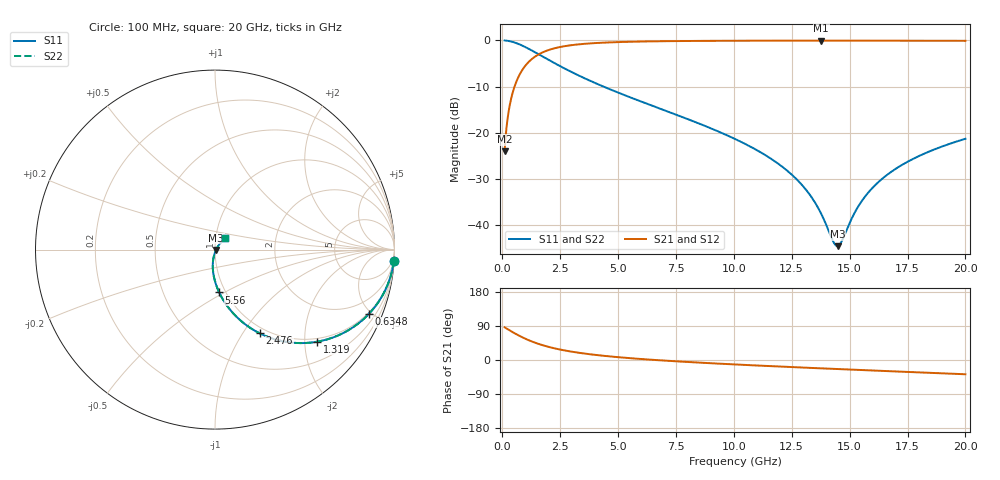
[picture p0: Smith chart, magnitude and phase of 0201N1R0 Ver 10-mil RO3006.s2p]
# GHz S MA R 50
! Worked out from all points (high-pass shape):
!   1601 points, 100 MHz to 20 GHz, reference 50 ohm
!   highest |S21| = -0.05 dB at 13.77 GHz (marker M1); lowest = -24.0 dB at 100 MHz (marker M2)
!   |S21| within 3 dB of the highest: 1.563 GHz to end of sweep
!   lowest |S11| = -44.6 dB at 14.48 GHz (marker M3), VSWR 1.01, Z = 50.5 - j0.238 ohm
!   |S11| at or under -10 dB: 4.364 GHz to end of sweep
!   |S22| runs from -44.6 to 0.0 dB; largest |S21 - S12| = 0
!   S11 on the Smith chart (normalised r, x): 100 MHz: 1, -30; 634.8 MHz: 0.92, -4.78; 1.319 GHz: 0.92, -2.29; 2.476 GHz: 0.92, -1.19; 5.56 GHz: 0.93, -0.47; 20 GHz: 1.11, +0.14
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0.1  0.998 -3.8  0.06274 86.2  0.06274 86.2  0.998 -3.8
0.3363125  0.9782 -12.5  0.2069 77.5  0.2069 77.5  0.9782 -12.5
0.6348125  0.9282 -22.8  0.3711 67.1  0.3711 67.1  0.9282 -22.8
0.9333125  0.8611 -32.0  0.5071 57.9  0.5071 57.9  0.8611 -32.0
1.318875  0.7666 -42.0  0.6403 47.8  0.6403 47.8  0.7666 -42.0
1.878562  0.6393 -53.2  0.7666 36.6  0.7666 36.6  0.6393 -53.2
2.475563  0.5292 -61.9  0.8457 27.8  0.8457 27.8  0.5292 -61.9
3.420812  0.4028 -71.5  0.9119 18.1  0.9119 18.1  0.4028 -71.5
5.560062  0.2396 -84.4  0.9667 4.6  0.9667 4.6  0.2396 -84.4
6.741625  0.185 -89.2  0.9782 -0.5  0.9782 -0.5  0.185 -89.2
10.05  0.08556 -98.4  0.991 -11.8  0.991 -11.8  0.08556 -98.4
12.06488  0.04327 -100.2  0.9933 -17.5  0.9933 -17.5  0.04327 -100.2
13.37081  0.01976 -94.2  0.9938 -21.0  0.9938 -21.0  0.01976 -94.2
13.76881  0.0133 -86.3  0.9938 -22.0  0.9938 -22.0  0.0133 -86.3
14.27875  0.006727 -52.7  0.9938 -23.4  0.9938 -23.4  0.006727 -52.7
14.47775  0.0059 -23.5  0.9937 -23.9  0.9937 -23.9  0.0059 -23.5
14.65188  0.006614 2.0  0.9937 -24.3  0.9937 -24.3  0.006614 2.0
15.14937  0.01261 35.9  0.9935 -25.6  0.9935 -25.6  0.01261 35.9
15.55981  0.01871 44.4  0.9934 -26.6  0.9934 -26.6  0.01871 44.4
16.69162  0.03607 50.5  0.9927 -29.5  0.9927 -29.5  0.03607 50.5
18.12194  0.05779 50.5  0.9914 -33.0  0.9914 -33.0  0.05779 50.5
20  0.08594 47.8  0.989 -37.6  0.989 -37.6  0.08594 47.8
